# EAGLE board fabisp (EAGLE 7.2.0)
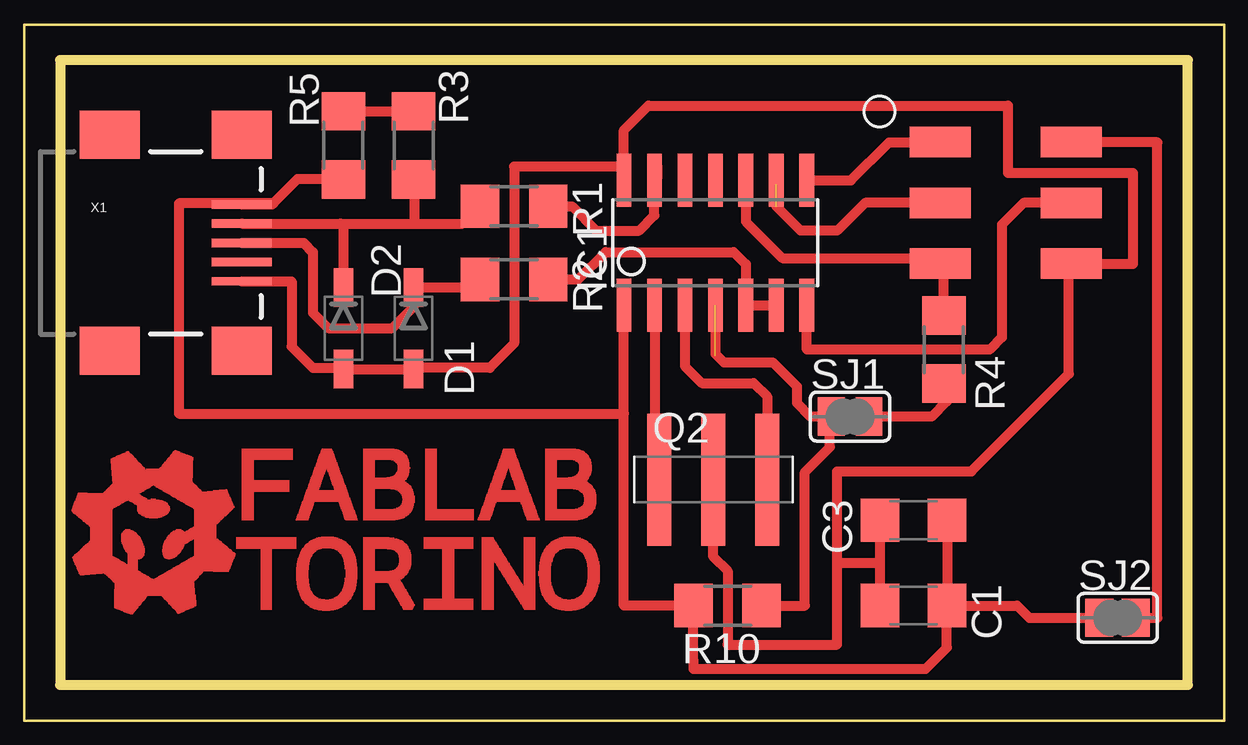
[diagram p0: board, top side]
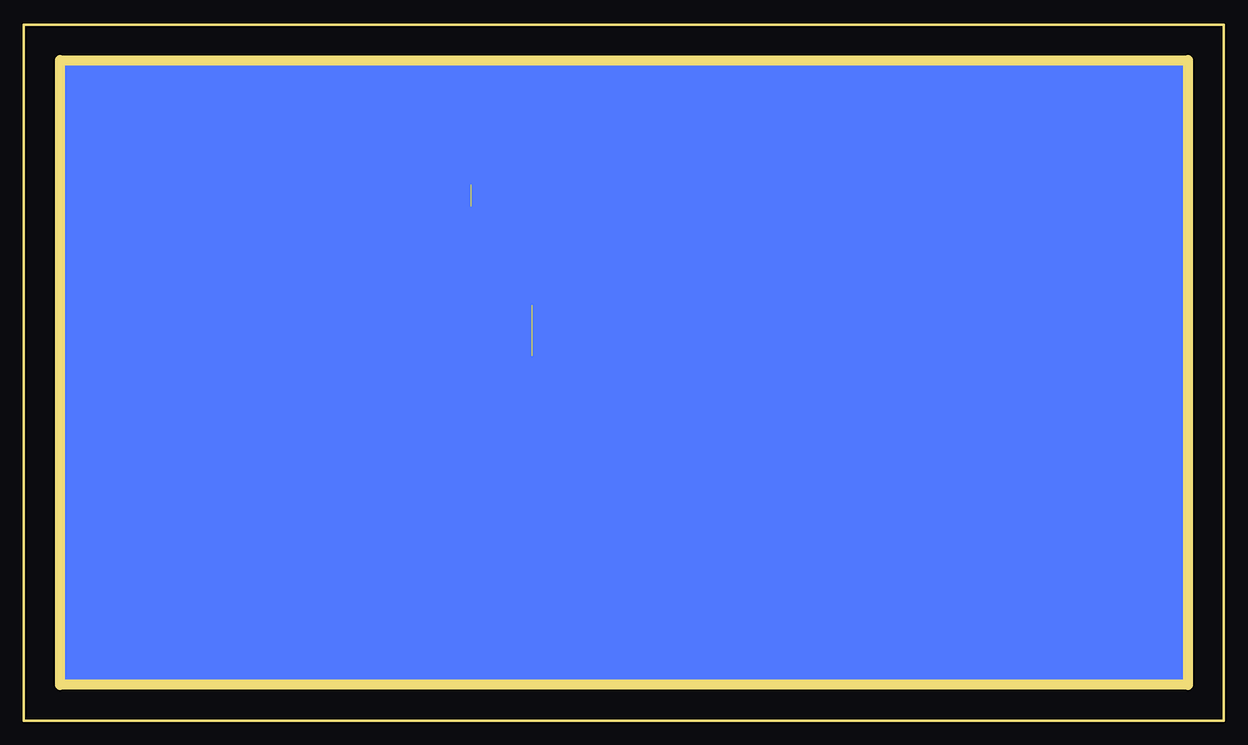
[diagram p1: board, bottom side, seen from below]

Size 46.99 x 26.04 mm. Coordinates in mm from the lower left corner, seen from the top.
Outline: 0,0 46.99,0 46.99,26.04 0,26.04 0,0
Copper layers (1*16): Top 0.035mm / dielectric 1.5mm / Bottom 0.035mm
Design rules "default *": minimum track width 12mil, minimum drill 24mil, track to track 17mil, track to pad 16mil, pad to pad 16mil, via to via 16mil, smd to smd 0mil, copper to edge 17mil, drill to drill 8mil, minimum pad ring 10mil, minimum via ring 8mil, stop-mask expansion 4mil, vias tented up to drill 0mil, thermal gap 10mil
Milling: 4 lines

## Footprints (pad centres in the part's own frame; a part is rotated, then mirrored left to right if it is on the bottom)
C1206 = smd 1.6 x 1.8: 1 -1.4,0; 2 1.4,0
SOD123 = smd 1.6 x 0.8: ANODE 1.7,0; CATHODE -1.7,0
SOIC14 = smd 0.61 x 2.21: 1 -3.81,-2.603; 2 -2.54,-2.603; 3 -1.27,-2.603; 4 0,-2.603; 5 1.27,-2.603; 6 2.54,-2.603; 7 3.81,-2.603; 8 3.81,2.603; 9 2.54,2.603; 10 1.27,2.603; 11 0,2.603; 12 -1.27,2.603; 13 -2.54,2.603; 14 -3.81,2.603
CSTCR6M = smd 1 x 5.5: 1 -2.25,0; 2 0,0; 3 2.25,0
R1206 = smd 1.6 x 1.803: 1 -1.422,0; 2 1.422,0
SJFAB = smd 1.118 x 1.6: 1 -0.787,0; 2 0.787,0
SJ = smd 1.168 x 1.6: 1 -0.762,0; 2 0.762,0
2X3_SMD = smd 2.54 x 1.27: 1 -2.54,2.54; 2 2.92,2.54; 3 -2.54,0; 4 2.92,0; 5 -2.54,-2.54; 6 2.92,-2.54
USB_MINIB = smd 2.5 x 0.35: D+ 3.77,0; D- 3.77,0.8; GND 3.77,-1.6; ID 3.77,-0.8; VBUS 3.77,1.6 | smd 2.5 x 2: GND@1 -1.73,-4.5; GND@2 -1.73,4.5; GND@3 3.77,4.5; GND@4 3.77,-4.5

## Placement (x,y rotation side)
C1  0.1uF  [C1206]  35.56,3.3 180 top
C3  10uF  [C1206]  35.56,6.86 180 top
D1  3.3V  [SOD123]  14.73,14.86 270 top
D2  3.3V  [SOD123]  11.81,14.86 270 top
IC1  ATTINY24/44/84-SSU  [SOIC14]  27.3,18.41 0 top
Q2  CSTCR6M00G53Z  [CSTCR6M]  27.22,8.55 0 top
R1  49  [R1206]  18.92,19.94 0 top
R2  49  [R1206]  18.92,16.89 0 top
R3  1K  [R1206]  14.73,22.48 90 top
R4  0  [R1206]  36.83,13.97 90 top
R5  499  [R1206]  11.81,22.48 270 top
R10  10K  [R1206]  27.81,3.3 180 top
SJ1  SJFAB  [SJFAB]  32.92,11.18 0 top
SJ2  [SJ]  44.07,2.79 0 top
U$1  2X3HEADER  [2X3_SMD]  39.22,20.09 0 top
X1  USB_MINIB  [USB_MINIB]  3.81,18.41 0 top

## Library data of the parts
C1 R1-R3 R10 = rcl-ez
C3 R4 R5 = rcl
D1 D2 = ng
IC1 = attiny24_44_84
Q2 = FablabTorino; MPN: CSTCR6M00G53-R0; OC_FARNELL: 1170434; OC_NEWARK: 25M8759
SJ1 U$1 X1 = mellis
SJ2 = jumper

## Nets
D+: IC1.5 IC1.6 R2.2
D-: IC1.13 R1.2
GND: C1.2 C3.2 D1.ANODE D2.ANODE IC1.14 Q2.2 U$1.6 X1.GND
MISO: IC1.8 U$1.1
MOSI: IC1.7 U$1.4
N$1: D2.CATHODE R1.1 R3.1 X1.D-
N$2: D1.CATHODE R2.1 X1.D+
N$3: R4.1 SJ1.2
N$4: IC1.2 Q2.1
N$5: IC1.3 Q2.3
N$6: R3.2 R5.1
RESET: IC1.4 R10.1 SJ1.1
RST: IC1.10 R4.2 U$1.5
SCK: IC1.9 U$1.3
VCC: C1.1 C3.1 IC1.1 R5.2 R10.2 SJ2.1 X1.VBUS
VCC': SJ2.2 U$1.2

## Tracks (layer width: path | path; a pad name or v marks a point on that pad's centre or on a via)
D+
  Top 0.406: R2.2 21.59,16.89 22.73,18.03 28.07,18.03 28.57,17.53 IC1.5 IC1.6
D-
  Top 0.406: R1.2 21.34,19.94 22.35,18.92 24.13,18.92 24.77,19.56 IC1.13 | IC1.13 24.77,21.46 24.89,21.59 24.89,21.14 IC1.13
GND
  Top 0.406: X1.GND 9.65,16.82 9.65,14.1 10.54,13.21 11.76,13.21 D2.ANODE | 11.81,13.08 D2.ANODE | D2.ANODE D1.ANODE 14.78,13.21 17.91,13.21 18.92,14.22 18.92,21.59 23.5,21.59 IC1.14 23.5,23.11 24.51,24.13 39.5,24.13 39.5,21.34 44.7,21.34 44.7,17.53 42.14,17.53 U$1.6 | 42.16,17.53 U$1.6 | C3.2 34.16,5.08 | 34.16,5.08 C1.2 | 32.38,5.08 34.16,5.08 | 32.38,5.08 32.38,8.89 37.97,8.89 42.04,12.95 42.04,17.44 U$1.6 | Q2.2 27.2,8.55 27.2,5.36 27.81,4.75 27.81,1.68 32.38,1.68 32.38,5.08
MISO
  Top 0.406: IC1.8 32.96,21.02 34.54,22.61 36.66,22.61 U$1.1
MOSI
  Top 0.406: U$1.4 40.15,20.09 39.24,19.18 39.24,14.48 38.73,13.97 31.11,13.97 IC1.7
N$1
  Top 0.406: D2.CATHODE 11.81,19.09 11.68,19.21 | 17.5,20.04 R1.1 16.78,19.21 14.76,19.21 | X1.D- 11.68,19.21 | 11.68,19.21 14.76,19.21 | R3.1 14.76,21.06 14.76,19.21
N$2
  Top 0.406: 17.14,17.02 17.27,16.89 R2.1 17.17,16.56 D1.CATHODE 14.73,15.75 13.84,14.86 11.18,14.86 10.54,15.49 10.54,18.03 10.16,18.41 X1.D+
N$3
  Top 0.406: R4.1 36.96,12.42 36.96,11.81 36.32,11.18 SJ1.2
N$4
  Top 0.406: IC1.2 24.72,15.77 24.79,15.77 24.79,8.73 Q2.1
N$5
  Top 0.406: IC1.3 26.04,13.28 26.75,12.57 28.91,12.57 29.46,12.01 Q2.3
N$6
  Top 0.406: R5.1 R3.2
RESET  (1 unrouted)
  Top 0.406: R10.1 31.04,3.3 31.04,8.87 32.08,9.91 32.08,11.12 SJ1.1 31.27,11.18 30.71,11.73 30.71,12.42 29.69,13.44 27.66,13.44 27.3,13.79 IC1.4
RST
  Top 0.406: IC1.10 28.57,19.3 30.1,17.78 36.45,17.78 U$1.5 36.83,17.4 R4.2
SCK  (1 unrouted)
  Top 0.406: U$1.3 33.55,20.09 32.38,18.92 30.86,18.92 29.84,19.94 | IC1.9 29.84,20.83
VCC
  Top 0.406: X1.VBUS 8.84,20.02 8.89,20.07 | 9.88,21.06 9.91,21.08 11.79,21.08 R5.2 9.88,21.06 | C1.1 39.88,3.3 40.39,2.79 SJ2.1 | C3.1 C1.1 | 23.5,11.3 23.5,3.3 R10.2 26.39,1.02 | 23.5,11.3 IC1.1 | 9.88,21.06 8.89,20.07 | 8.89,20.07 4.95,20.07 4.95,11.3 23.5,11.3 | 26.39,1.02 | 26.39,1.02 26.39,0.66 36.07,0.66 36.96,1.55 C1.1
VCC'
  Top 0.406: SJ2.2 45.72,2.79 45.72,22.61 42.14,22.61 U$1.2
(copper drawn outside any net)
  shapes: Bottom area x1, Top area x2926

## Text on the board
tKeepout: VTG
